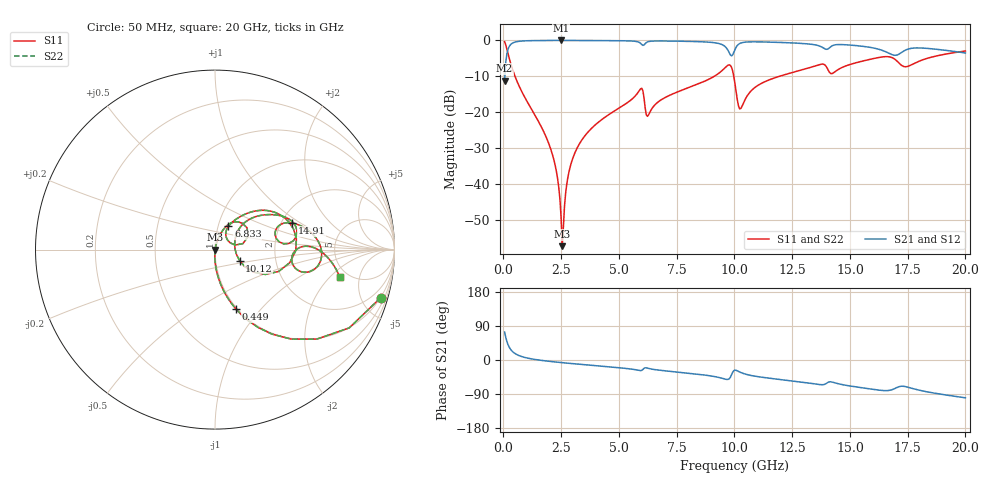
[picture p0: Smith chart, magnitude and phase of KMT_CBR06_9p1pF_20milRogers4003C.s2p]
! Data measured by Modelithics Inc. support@modelithics.com 813-866-6335
! KEMET CBR0603 9.1pF, Pad Width= 0.851mm, Pad Length= 0.64mm, Pad Gap= 0.62mm, 20mil Rogers 4003C substrate Data, January 2022
# hz S ma R 50
! 2 Port Network Data from SP1.SP block
! freq  magS11  angS11  magS21  angS21  magS12  angS12  magS22  angS22
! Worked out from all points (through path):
!   401 points, 50 MHz to 20 GHz, reference 50 ohm
!   highest |S21| = -0.01 dB at 2.494 GHz (marker M1); lowest = -11.2 dB at 50 MHz (marker M2)
!   group delay of S21, straight-line fit = 14.5 ps
!   lowest |S11| = -57.2 dB at 2.544 GHz (marker M3), VSWR 1.00, Z = 50.1 - j0.0711 ohm
!   |S11| at or under -10 dB: 500.7 MHz to 9.122 GHz (8.622 GHz wide, 179 % of centre); 9.972 GHz to 11.94 GHz (1.967 GHz wide, 18 % of centre)
!   |S22| runs from -57.2 to -0.3 dB; largest |S21 - S12| = 0
!   S11 on the Smith chart (normalised r, x): 50 MHz: 0.99, -6.88; 449 MHz: 0.99, -0.74; 6.833 GHz: 1.12, +0.30; 10.12 GHz: 1.31, -0.16; 14.91 GHz: 2.27, +0.85; 20 GHz: 4.23, -2.65
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5e7  0.9608 -16.2  0.277 73.8  0.277 73.8  0.9608 -16.2
4.49e8  0.3507 -70.6  0.9357 19.3  0.9357 19.3  0.3507 -70.6
2.045e9  0.03097 -91.8  0.9983 -3.9  0.9983 -3.9  0.03097 -91.8
2.294375e9  0.01496 -90.9  0.9986 -5.5  0.9986 -5.5  0.01496 -90.9
2.493875e9  0.003547 -76.2  0.9987 -6.7  0.9987 -6.7  0.003547 -76.2
2.54375e9  0.001376 -31.0  0.9987 -7.0  0.9987 -7.0  0.001376 -31.0
2.892875e9  0.01764 76.6  0.9984 -9.0  0.9984 -9.0  0.01764 76.6
3.391625e9  0.04114 76.2  0.9976 -11.8  0.9976 -11.8  0.04114 76.2
5.93525e9  0.2118 43.8  0.9132 -28.0  0.9132 -28.0  0.2118 43.8
6.2345e9  0.08792 37.5  0.9517 -21.6  0.9517 -21.6  0.08792 37.5
6.73325e9  0.1424 60.1  0.9819 -26.8  0.9819 -26.8  0.1424 60.1
6.833e9  0.1496 60.0  0.9818 -27.5  0.9818 -27.5  0.1496 60.0
9.72575e9  0.4524 14.5  0.724 -51.1  0.724 -51.1  0.4524 14.5
1.0025e10  0.2487 -30.3  0.7513 -26.7  0.7513 -26.7  0.2487 -30.3
1.012475e10  0.1496 -24.0  0.8504 -28.5  0.8504 -28.5  0.1496 -24.0
1.027438e10  0.1128 13.6  0.9188 -32.9  0.9188 -32.9  0.1128 13.6
1.092275e10  0.2261 42.3  0.9555 -43.0  0.9555 -43.0  0.2261 42.3
1.336662e10  0.429 25.0  0.8807 -62.0  0.8807 -62.0  0.429 25.0
1.491275e10  0.4527 19.1  0.8661 -67.6  0.8661 -67.6  0.4527 19.1
1.670825e10  0.5908 -6.3  0.6587 -80.2  0.6587 -80.2  0.5908 -6.3
1.74065e10  0.4302 -6.2  0.7332 -70.2  0.7332 -70.2  0.4302 -6.2
2e10  0.7126 -12.5  0.668 -99.8  0.668 -99.8  0.7126 -12.5
